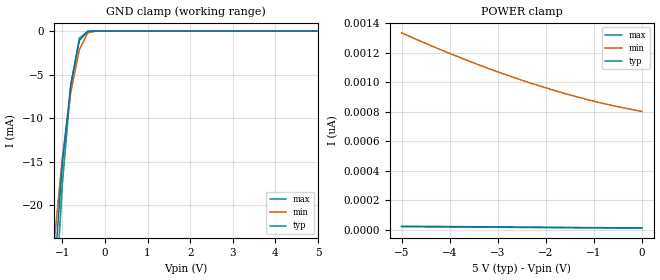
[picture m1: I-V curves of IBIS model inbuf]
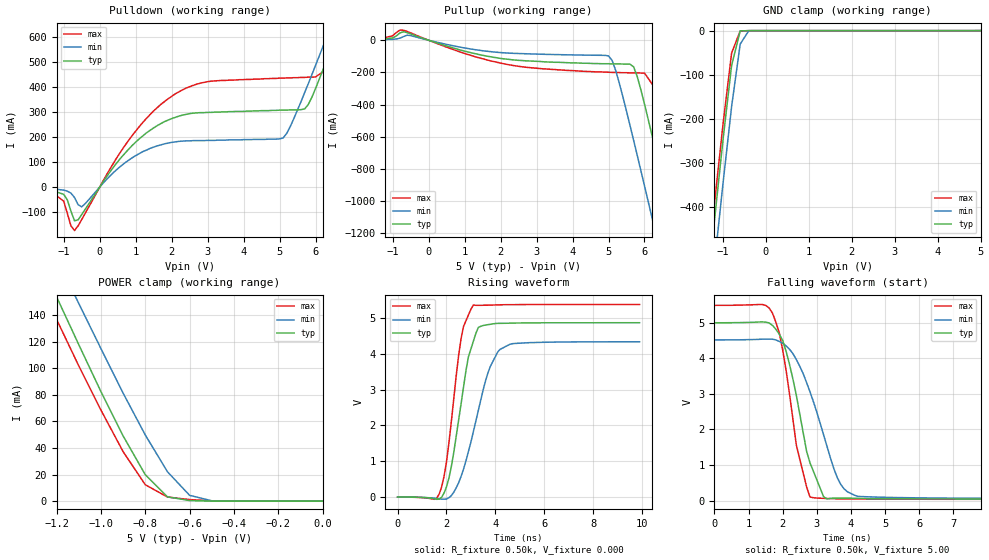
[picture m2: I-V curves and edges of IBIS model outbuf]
| IBIS file 40806k.ibs created by s2ibis2 version 1.0
| North Carolina State University Electronics Research Laboratory  1995
[IBIS ver]   2.1
[File name]   40806k.ibs
[File Rev]   0.1
[Date]   Thursday, May 29, 1997
[Source]   IDT
[Notes]   1. Temp typ=25C, min=100C, max=0C 2. Ramp rates based on 500
   ohm load
[Copyright]   Copyright 1997, Integrated Device Technology, Inc.
[Disclaimer] Integrated Device Technology, Inc. ("IDT") hereby grants the
   user of this IBIS model a non-exclusive, nontransferable
   license to use this IBIS model under the following terms.
   The user is granted this license only to use the IBIS model
   and is not granted rights to sell, copy (except as needed to
   run the IBIS model), rent, lease or sub-license the IBIS model
   in whole or in part, or in modified form to anyone.
   The User may modify the IBIS model to suit its specific
   applications, but rights to derivative works and such
   modifications shall belong to IDT.
   This IBIS model is provided on an "AS IS" basis and IDT
   makes absolutely no warranty with respect to the information
   contained herein. IDT DISCLAIMS AND CUSTOMER WAIVES ALL
   WARRANTIES, EXPRESS AND IMPLIED, INCLUDING WARRANTIES OF
   MERCHANTABILITY AND FITNESS FOR A PARTICULAR PURPOSE. THE
   ENTIRE RISK AS TO QUALITY AND PERFORMANCE IS WITH THE
   USER ACCORDINGLY, IN NO EVENT SHALL IDT BE LIABLE
   FOR ANY DIRECT OR INDIRECT DAMAGES, WHETHER IN CONTRACT OR
   TORT, INCLUDING ANY LOST PROFITS OR OTHER INCIDENTAL,
   CONSEQUENTIAL, EXEMPLARY, OR PUNITIVE DAMAGES ARISING OUT OF
   THE USE OR APPLICATION OF THE IBIS model.  Further, IDT
   reserves the right to make changes without notice to any
   product herein to improve reliability, function, or design.
   IDT does not convey any license under patent rights or
   any other intellectual property rights, including those of
   third parties. IDT is not obligated to provide maintenance
   or support for the licensed IBIS model.
|   Component IDT49FCT806/A
[Component]   IDT49FCT806/A
[Manufacturer]   Integrated Device Technology Inc.
[Package]
| Following package parameters are for D20-1(CDIP), P20-1(DPIP) packages
|[Package]
|| variable   typ   min   max
|R_pkg   40.00m   30.00m   50.00m
|L_pkg   7.00nH   4.00nH   10.00nH
|C_pkg   0.60pF   0.50pF   0.70pF
| Following package parameters are for SO20-6(EIAJ), SO20-2(SOIC) packages
|[Package]
|| variable   typ   min   max
|R_pkg   25.00m   20.00m   30.00m
|L_pkg   3.50nH   2.10nH   6.50nH
|C_pkg   0.40pF   0.35pF   0.60pF
| Following package parameters are for SO20-8(QSOP), SO20-7(SSOP) packages
| variable   typ   min   max
R_pkg   20.00m   15.00m   25.00m
L_pkg   3.00nH   2.00nH   4.00nH
C_pkg   0.30pF   0.26pF   0.34pF
[Pin]  signal_name   model_name   R_pin   L_pin   C_pin
1   VCCA   POWER
2   OA1   outbuf
3   OA2   outbuf
4   OA3   outbuf
5   GNDA   GND
6   OA4   outbuf
7   OA5   outbuf
8   GNDQ   GND
9   OEAB   inbuf
10   INA   inbuf
11   INB   inbuf
12   OEBB   inbuf
13   MON   outbuf
14   OB5   outbuf
15   OB4   outbuf
16   GNDB   GND
17   OB3   outbuf
18   OB2   outbuf
19   OB1   outbuf
20   VCCB   POWER
| Models and submodels in the file (2): inbuf (Input), outbuf (3-state)
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| in   IN1   dummy_model
| oe   OE1   dummy_model
|   Model inbuf
[Model]   inbuf
Model_type   Input
Vinl =  0.800V
Vinh =  2.000V
C_comp   3.00pF   NA   NA
[Temperature Range]   25.00   100.00   0.000
[Voltage Range]   5.00V   4.50V   5.50V
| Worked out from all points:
|   GND clamp passes 1 mA (typ) near -0.59 V on its own axis
[GND_clamp]
| voltage   I(typ)   I(min)   I(max)
-5V       -67.15A    -63.94A    -68.24A
-1.2V     -28.45mA   -24.7mA    -34.05mA
-1V       -15.28mA   -14.53mA   -17.56mA
-800mV    -6.017mA   -6.948mA   -6.255mA
-600mV    -1.078mA   -2.117mA   -816uA
-400mV    -19.55uA   -178uA     -9.254uA
-200mV    -4.103nA   -287nA     -753pA
5V        12.62pA    835pA      10.26pA
[POWER_clamp]
| voltage   I(typ)   I(min)   I(max)
-5V       24.47pA    1.335nA    21.41pA
-4.3V     22.78pA    1.236nA    20pA
-3.6V     21.06pA    1.144nA    18.56pA
-3V       19.62pA    1.071nA    17.33pA
-2.3V     17.96pA    993pA      15.92pA
-1.7V     16.51pA    933pA      14.68pA
-1.1V     15.13pA    880pA      13.48pA
-600mV    13.99pA    842pA      12.44pA
0V        12.65pA    803pA      11.24pA
|   Model outbuf
[Model]   outbuf
Model_type   3-state
Polarity   Non-Inverting
Enable   Active-High
Vinl =  0.800V
Vinh =  2.000V
C_comp   3.00pF   NA   NA
[Temperature Range]   25.00   100.00   0.000
[Voltage Range]   5.00V   4.50V   5.50V
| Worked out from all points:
|   slope of the pulldown table from 0 to 0.75 V, typ, clamps not added: 5.24 ohm
|   slope of the pullup table from 0 to 0.75 V, typ, clamps not added: 14.3 ohm
|   GND clamp passes 1 mA (typ) near -0.60 V on its own axis
|   POWER clamp passes 1 mA (typ) near -0.62 V on its own axis
|   rising waveform, R_fixture 0.50k, V_fixture 0.000: 20-80 % time 663ps typ, 961ps min, 553ps max; typ from 0 V to 4.87 V
|   falling waveform, R_fixture 0.50k, V_fixture 5.00: 20-80 % time 660ps typ, 909ps min, 544ps max; typ from 5 V to 0.045 V
[Pulldown]
| voltage   I(typ)   I(min)   I(max)
-5V       -2mA       -1mA       -2mA
-1.4V     -9.7mA     -5.8mA     -13.4mA
-700mV    -135mA     -41.49mA   -174mA
-500mV    -110mA     -79.11mA   -130mA
900mV     166mA      117mA      206mA
2.3V      288mA      184mA      389mA
5.1V      308mA      197mA      436mA
5.7V      313mA      379mA      439mA
6.4V      540mA      633mA      480mA
6.8V      692mA      781mA      616mA
7.2V      845mA      929mA      761mA
10V       1.93A      1.977A     1.801A
[Pullup]
| voltage   I(typ)   I(min)   I(max)
-5V       0A         0A         1mA
-700mV    53.19mA    22.65mA    62.45mA
2.1V      -116mA     -78.21mA   -147mA
5V        -146mA     -97.26mA   -199mA
5.2V      -147mA     -188mA     -200mA
5.7V      -166mA     -624mA     -203mA
6V        -396mA     -905mA     -204mA
6.4V      -768mA     -1.285A    -332mA
6.8V      -1.15A     -1.668A    -691mA
7.2V      -1.536A    -2.053A    -1.067A
7.6V      -1.924A    -2.439A    -1.448A
10V       -4.261A    -4.764A    -3.75A
[GND_clamp]
| voltage   I(typ)   I(min)   I(max)
-5V       -4.127A    -4.193A    -4.048A
-1.4V     -619mA     -716mA     -579mA
-1.2V     -431mA     -529mA     -393mA
-1V       -247mA     -346mA     -212mA
-800mV    -78.83mA   -172mA     -50.8mA
-600mV    -706uA     -30.53mA   -739uA
-400mV    -302nA     -159uA     -17.95nA
5V        402fA      264uA      124fA
[POWER_clamp]
| voltage   I(typ)   I(min)   I(max)
-5V       1.606A     1.587A     1.529A
-1.3V     191mA      220mA      172mA
-1.2V     154mA      184mA      137mA
-1.1V     118mA      149mA      102mA
-1V       82.58mA    115mA      68.66mA
-900mV    49.17mA    81.42mA    37.36mA
-800mV    19.95mA    49.86mA    12.36mA
-700mV    3.23mA     22.14mA    3.104mA
-600mV    417uA      4.37mA     1.165mA
-500mV    2.462uA    264uA      211uA
0V        402fA      2.846nA    160fA
[Ramp]
| variable   typ   min   max
dV/dt_r   2.92/0.66n   2.60/0.96n   3.23/0.55n
dV/dt_f   2.97/0.66n   2.67/0.91n   3.27/0.55n
R_load = 0.50k
[Rising Waveform]
R_fixture = 0.50k
V_fixture = 0.000
| time   V(typ)   V(min)   V(max)
0s        0V         0V         0V
1.7ns     -57.59mV   -48.53mV   82.7mV
2.1ns     528mV      -19.14mV   1.512V
2.6ns     2.614V     583mV      4.435V
2.9ns     3.92V      1.276V     5.086V
3.1ns     4.35V      1.824V     5.361V
3.3ns     4.734V     2.408V     5.354V
3.7ns     4.814V     3.475V     5.358V
4.2ns     4.851V     4.127V     5.368V
9.9ns     4.868V     4.336V     5.377V
[Falling Waveform]
R_fixture = 0.50k
V_fixture = 5.00
| time   V(typ)   V(min)   V(max)
0s        5V         4.517V     5.488V
1.7ns     4.926V     4.537V     5.27V
1.9ns     4.677V     4.476V     4.713V
2.1ns     4.197V     4.348V     3.66V
2.4ns     2.96V      3.966V     1.562V
2.8ns     1.062V     3.059V     103mV
3.2ns     108mV      1.845V     65.39mV
3.7ns     70.9mV     459mV      52.79mV
4.1ns     67.51mV    155mV      49.94mV
9.9ns     45.03mV    62.61mV    37.9mV
